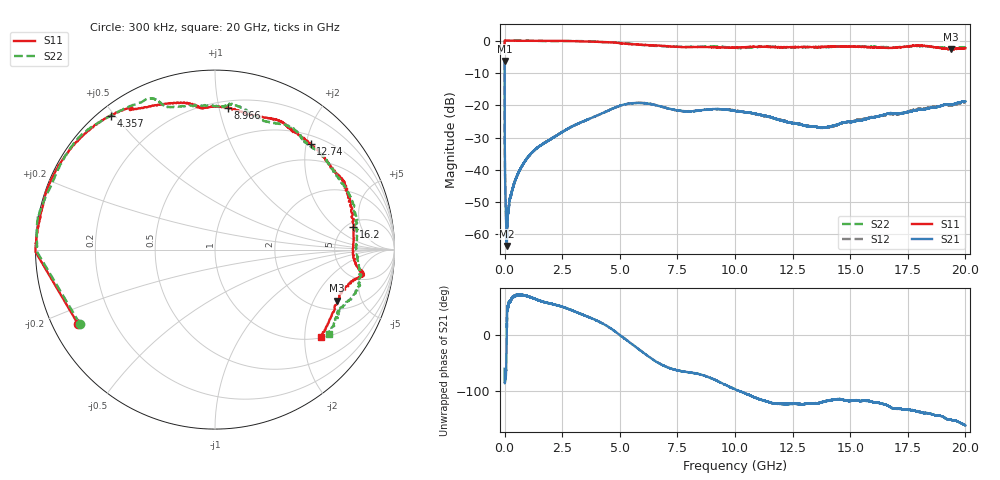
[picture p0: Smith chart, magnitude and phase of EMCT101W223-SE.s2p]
!EMCT101W223
!Johanson Technology Inc.
!www.johansontechnology.com
!Test Board Conditions:
!Substrate Type  RO4350B
!Substrate Thickness  10 mil
!Substrate Dk  3.66
!TL Type: GCPW
!TL Trace Width  22 mil
!TL Gap  14 mil
!PART MODE SINGLE ENDED (AKA BYPASS)
!DUT TOPOLOGY	SERIES-SHUNT
# MHz S  dB  R 50
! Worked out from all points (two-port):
!   20001 points, 300 kHz to 20 GHz, reference 50 ohm
!   highest |S21| = -6.32 dB at 300 kHz (marker M1); lowest = -63.6 dB at 94.3 MHz (marker M2)
!   |S21| within 3 dB of the highest: start of sweep to 561.8 kHz
!   lowest |S11| = -2.7 dB at 19.39 GHz (marker M3), VSWR 6.54, Z = 125 - j154 ohm
!   |S11| at or under -10 dB: nowhere
!   |S22| runs from -2.3 to 0.0 dB; largest |S21 - S12| = 0.0056
!   S11 on the Smith chart (normalised r, x): 300 kHz: 0.07, -0.25; 4.357 GHz: 0.03, +0.49; 8.966 GHz: 0.25, +1.07; 12.74 GHz: 0.65, +2.08; 16.2 GHz: 5.73, +3.68; 20 GHz: 1.02, -2.41
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0.3  -1.23 -151.3  -6.32 -60.3  -6.32 -60.3  -1.32 -151.2
94.299  -0.01 178.9  -63.59 10.0  -63.18 1.5  -0.07 179.2
113.298  -0.01 178.7  -59.03 41.3  -58.65 41.9  -0.07 179.0
150.298  -0.03 178.2  -53.40 50.6  -53.54 51.3  -0.06 178.8
276.296  -0.03 176.8  -48.13 62.5  -47.87 60.9  -0.06 177.2
472.293  -0.04 174.6  -43.09 70.3  -43.06 70.6  -0.03 175.1
1115.283  -0.06 167.5  -35.22 67.7  -35.26 67.6  -0.02 167.8
3334.25  -0.23 139.3  -25.23 37.2  -25.26 37.4  -0.17 139.1
4357.235  -0.48 127.9  -22.12 18.2  -22.13 18.2  -0.48 127.6
5100.224  -0.86 120.3  -19.93 -3.2  -20.00 -3.0  -0.75 113.7
6667.2  -1.55 101.9  -20.20 -49.6  -20.16 -50.0  -1.68 105.0
7874.182  -2.03 95.0  -21.90 -65.8  -21.86 -65.7  -1.94 89.3
8966.166  -2.02 84.7  -21.25 -77.3  -21.31 -76.9  -1.77 83.5
10000.15  -2.18 72.3  -21.78 -97.0  -21.63 -96.9  -2.27 72.0
12739.11  -1.99 48.0  -25.84 -123.0  -25.73 -123.2  -2.08 45.4
13334.1  -2.02 38.5  -26.57 -122.2  -26.57 -122.5  -2.03 37.7
15168.07  -1.84 24.9  -25.05 -117.1  -24.84 -115.8  -1.82 17.6
16200.06  -2.14 9.2  -23.45 -121.1  -23.52 -122.2  -1.94 6.7
16667.05  -2.28 0.5  -22.51 -126.8  -22.79 -126.4  -2.08 1.8
18031.03  -1.64 -10.1  -21.34 -137.4  -21.11 -137.6  -1.73 -15.0
19385.01  -2.68 -22.8  -19.83 -151.5  -20.08 -153.0  -2.26 -27.9
20000  -2.32 -39.5  -18.79 -161.5  -18.99 -159.3  -2.05 -36.7
